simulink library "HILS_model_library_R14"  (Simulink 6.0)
undefined symbols (not defined in the file or in its folder): hilsmdl
libraries: simulink x47, simulink_extras x9, HILS_model_library x3
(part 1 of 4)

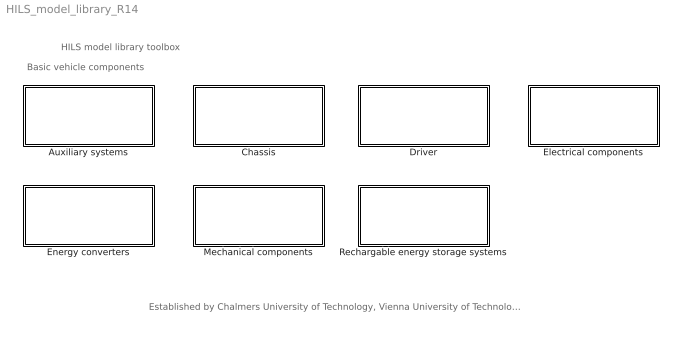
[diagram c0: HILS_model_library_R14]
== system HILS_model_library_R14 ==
  note: HILS model library toolbox
  note: Basic vehicle components
  note: Established by Chalmers University of Technology, Vienna University of Technology, Graz University of Technology, 2014
  Auxiliary systems : Subsystem
  Chassis : Subsystem
  Driver : Subsystem
  Electrical components : Subsystem
  Energy converters : Subsystem
  Mechanical components : Subsystem
  Rechargable energy storage systems : Subsystem

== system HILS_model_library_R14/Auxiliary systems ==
  Electrical auxiliary system : Subsystem
  Mechanical auxiliary system : Subsystem  mask{dat=hilsmdl.mechaux}
      mask prompts: dat "Elmotor parameter data name [struct]"

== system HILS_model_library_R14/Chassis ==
  Chassis : Subsystem  mask{dat=hilsmdl.chassis}
      mask prompts: dat "Chassis system parameter name [struct]"

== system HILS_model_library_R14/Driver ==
  Gearshift logics for manual transmission : Subsystem  mask{dat=hilsmdl.drivermanual.gearshiftmanual}
      mask prompts: dat "manual gearshift logics parameter name"
  Vehicle driver (Automatic) : Subsystem  mask{dat=hilsmdl.driverautomatic}
      mask prompts: dat "driver parameter name [struct]"
      mask help: Driver model
  Vehicle driver (Manual) : Subsystem  mask{dat=hilsmdl.drivermanual}
      mask prompts: dat "driver parameter name [struct]"
      mask help: Driver model
  Vehicle driver (Measured data) : Subsystem

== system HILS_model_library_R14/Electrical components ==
  DCDC converter : Subsystem  mask{dat=hilsmdl.dcdc}
      mask prompts: dat "DCDC parameter data name [struct]"

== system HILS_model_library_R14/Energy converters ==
  Electric machine : Subsystem  mask{dat=hilsmdl.elmachine}
      mask prompts: dat "Elmotor parameter data name [struct]"
  Hydraulic machine : Subsystem  mask{dat=hilsmdl.hydraulicmachine}
      mask prompts: dat "Hydraulic pump/motor parameter data [struct]"
  Internal Combustion Engine : Subsystem  mask{dat=hilsmdl.eng}
      mask prompts: dat "ICE parameter name [struct]"

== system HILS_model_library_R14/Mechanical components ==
  Clutch : Subsystem  mask{dat=hilsmdl.clutch}
      mask prompts: dat "Clutch system parameter name [struct]"
  Continuously variable transmission : Subsystem  mask{dat=hilsmdl.cvt}
      mask prompts: dat "Gearbox parameter data name [struct]"
  Final gear : Subsystem  mask{dat=hilsmdl.finalgear}
      mask prompts: dat "Mechanical gear parameter name [struct]"
  Mechanical connection : Subsystem  mask{dat=hilsmdl.mechconnection}
      mask prompts: dat "Mechanical gear parameter name [struct]"
  Retarder : Subsystem  mask{dat=hilsmdl.retarder}
      mask prompts: dat "Gearbox parameter data name [struct]"
  Spur gear : Subsystem  mask{dat=hilsmdl.spurgear}
      mask prompts: dat "Mechanical gear parameter name [struct]"
  Torque converter : Subsystem  mask{dat=hilsmdl.torqueconverter}
      mask prompts: dat "Torque converter parameter data name [struct]"
  Transmission : Subsystem  mask{dat=hilsmdl.transmission}
      mask prompts: dat "Gearbox parameter data name [struct]"

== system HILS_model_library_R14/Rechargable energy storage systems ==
  Accumulator : Subsystem  mask{dat=hilsmdl.accumulator}
      mask prompts: dat "RESS system parameter name [struct]"
  Battery : Subsystem  mask{dat=hilsmdl.battery}
      mask prompts: dat "RESS system parameter name [struct]"
  Flywheel : Subsystem  mask{dat=hilsmdl.flywheel}
      mask prompts: dat "Mechanical gear parameter name [struct]"
  Super Capacitor : Subsystem  mask{dat=hilsmdl.supercapacitor}
      mask prompts: dat "RESS system parameter name [struct]"

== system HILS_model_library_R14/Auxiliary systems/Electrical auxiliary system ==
  cmd : Inport
  elec in [V] : Inport  Port=2
  Model Info : simulink/Model-Wide Utilities/Model Info  InitialBlockCM=None  BlockCM=None  Frame=on  DisplayStringWithTags=|  HorizontalTextAlignment=Left  LeftAlignmentValue=0.02  SourceBlockDiagram=HILS_model_library_R14  TagMaxNumber=20
      | This model level is fixed. Place parameters in the
      | system mask on the top level. The parameter is
      | a structure specified according to GTR No XXX.
  auxiliary system : Subsystem
  local controller : Subsystem
  sensor : Outport
  elec fb out [A] : Outport  Port=2
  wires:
  local controller/1(sensor out) -> sensor/1
  auxiliary system/2(el fb out [A]) -> elec fb out [A]/1
  cmd/1 -> local controller/1(cmd in)
  elec in [V]/1 -> auxiliary system/2(el in [V])
  auxiliary system/1(sensor out) -> local controller/2(sensor in)
  local controller/2(ctrl out) -> auxiliary system/1(ctrl in)

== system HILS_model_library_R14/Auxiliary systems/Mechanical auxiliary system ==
  cmd : Inport
  mech fb in [rad/s] : Inport  Port=2
  Model Info : simulink/Model-Wide Utilities/Model Info  InitialBlockCM=None  BlockCM=None  Frame=on  DisplayStringWithTags=|  HorizontalTextAlignment=Left  LeftAlignmentValue=0.02  SourceBlockDiagram=HILS_model_library_R14  TagMaxNumber=20
      | This model level is fixed. Place parameters in the
      | system mask on the top level. The parameter is
      | a structure specified according to GTR No XXX.
  auxiliary system : Subsystem
  local controller : Subsystem
  sensor : Outport
  mech out [Nm] : Outport  Port=2
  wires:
  local controller/2(ctrl out) -> auxiliary system/1(ctrl in)
  auxiliary system/1(sensor out) -> local controller/2(sensor in)
  mech fb in [rad/s]/1 -> auxiliary system/2(mech fb in [rad/s])
  cmd/1 -> local controller/1(cmd in)
  auxiliary system/2(mech out [Nm]) -> mech out [Nm]/1
  local controller/1(sensor out) -> sensor/1

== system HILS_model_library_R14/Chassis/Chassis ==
  cmd : Inport
  mech in [Nm] : Inport  Port=2
  Model Info : simulink/Model-Wide Utilities/Model Info  InitialBlockCM=None  BlockCM=None  Frame=on  DisplayStringWithTags=|  HorizontalTextAlignment=Left  LeftAlignmentValue=0.02  SourceBlockDiagram=HILS_model_library_R14  TagMaxNumber=20
      | This model level is fixed. Place parameters in the
      | system mask on the top level. The parameter is
      | a structure specified according to GTR No XXX.
  chassis : Subsystem
  local controller : Subsystem
  sensor : Outport
  mech fb out [rad/s] : Outport  Port=2
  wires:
  cmd/1 -> local controller/1(cmd in)
  local controller/1(sensor out) -> sensor/1
  chassis/1(sensor out) -> local controller/2(sensor in)
  mech in [Nm]/1 -> chassis/2(mech in [Nm])
  chassis/2(mech fb out [rad/s]) -> mech fb out [rad/s]/1
  local controller/2(ctrl) -> chassis/1(ctrl)

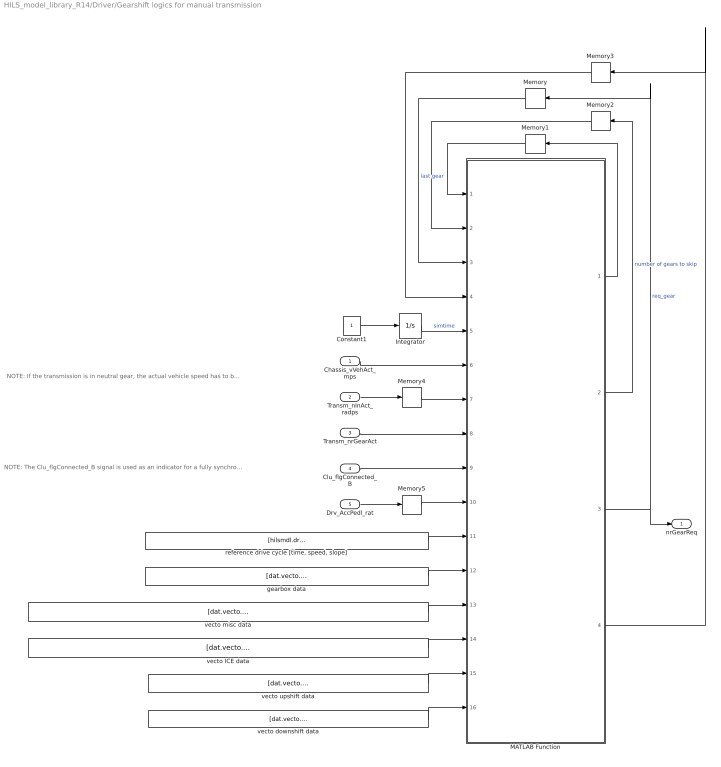
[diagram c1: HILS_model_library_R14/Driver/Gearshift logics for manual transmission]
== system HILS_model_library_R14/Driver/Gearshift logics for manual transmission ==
  note: NOTE: If the transmission is in neutral gear, the actual vehicle speed has to be zero (no rolling of the vehicle, application of brake necessary) for a correct engagement of the starting gear. Otherwise a time delay can occur until the starting gear is engaged.
  note: NOTE: The Clu_flgConnected_B signal is used as an indicator for a fully synchronized and connected drivetrain. It is involved in triggering upcoming gear shift events. Ensure that this signal becomes active only if the entire drivetrain runs on fully synchronized speeds.
  Chassis_vVehAct_mps : Inport
  Transm_nInAct_radps : Inport  Port=2
  Transm_nrGearAct : Inport  Port=3
  Clu_flgConnected_B : Inport  Port=4
  Drv_AccPedl_rat : Inport  Port=5
  Constant1 : Constant
  Integrator : Integrator
  MATLAB Function : Stateflow chart  TreatAsAtomicUnit=on
  Memory{,1..3} (4 alike) : Memory  Orientation=left
  Memory4 : Memory
  Memory5 : Memory
  gearbox data : Constant  Value=[dat.vecto.gear.number.vec; dat.vecto.gear.ratio.vec; dat.vecto.gear.efficiency.vec]
  "reference drive cycle [time, speed, slope]" : Constant  Value=[hilsmdl.drivecycle.time.vec, hilsmdl.drivecycle.speed.vec,hilsmdl.drivecycle.slope.vec]
  vecto ICE data : Constant  Value=[dat.vecto.ICE.maxtorque_speed.vec; dat.vecto.ICE.maxtorque_torque.vec; dat.vecto.ICE.maxtorque_friction.vec]
  vecto downshift data : Constant  Value=[dat.vecto.downshift_torque.vec; dat.vecto.downshift_speed.vec]
  vecto misc data : Constant  Value=[dat.vecto.vehicle.mass.value, dat.vecto.fg.ratio.value, 0.95, dat.vecto.wheel.radius.value, dat.vecto.wheel.inertia.value, dat.vecto.wheel.rollingres.value, dat.vecto.aero.af.value, dat.vecto.aero.cd.value, 80, dat.vecto.ICE.ratedspeed.value, 30, 3, dat.vecto.clutchtime.value,dat.vecto.skipgears.value,30,dat.vecto.startgearengaged.value,dat.vecto.startgearactive.value]  VectorParams1D=off
  vecto upshift data : Constant  Value=[dat.vecto.upshift_torque.vec; dat.vecto.upshift_speed.vec]
  nrGearReq : Outport
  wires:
  Constant1/1 -> Integrator/1
  Chassis_vVehAct_mps/1 -> MATLAB Function/6(act_vehicle_speed)
  MATLAB Function/3(req_gear) -> Memory/1, nrGearReq/1  "req_gear"
  "reference drive cycle [time, speed, slope]"/1 -> MATLAB Function/11(ref_drive_cycle)
  Integrator/1 -> MATLAB Function/5(simtime)  "simtime"
  Memory/1 -> MATLAB Function/3(last_req_gear)  "last gear"
  Clu_flgConnected_B/1 -> MATLAB Function/9(clutches_locked)
  Memory1/1 -> MATLAB Function/1(indicator_in)
  Transm_nInAct_radps/1 -> Memory4/1
  vecto misc data/1 -> MATLAB Function/13(VectoMisc)
  gearbox data/1 -> MATLAB Function/12(gbx)
  vecto upshift data/1 -> MATLAB Function/15(VectoShiftUp)
  MATLAB Function/2(skip_nr) -> Memory2/1  "number of gears to skip"
  Memory2/1 -> MATLAB Function/2(skip_nr_in)
  vecto ICE data/1 -> MATLAB Function/14(VectoICE)
  vecto downshift data/1 -> MATLAB Function/16(VectoShiftDown)
  MATLAB Function/1(indicator) -> Memory1/1
  MATLAB Function/4(simtime_prev_out) -> Memory3/1
  Memory3/1 -> MATLAB Function/4(simtime_prev)
  Transm_nrGearAct/1 -> MATLAB Function/8(act_gear)
  Memory4/1 -> MATLAB Function/7(act_rotational_speed)
  Drv_AccPedl_rat/1 -> Memory5/1
  Memory5/1 -> MATLAB Function/10(acc_pedal)

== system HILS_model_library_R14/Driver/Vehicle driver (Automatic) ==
  sensor in : Inport
  Bus Creator3 : BusCreator  Inputs=5
  Bus Selector1 : BusSelector  OutputSignals=Chassis.Chassis_vVehAct_mps
  Driver RefSpeed : Subsystem
  Ground : Ground
  Ground1 : Ground
  driver cmd out : Outport
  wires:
  Ground1/1 -> Bus Creator3/5  "Drv_CluPedl_Rt"
  Ground/1 -> Bus Creator3/4  "Drv_nrGearReq"
  Bus Selector1/1 -> Driver RefSpeed/1(Chassis_vVehAct_mps)  "<Chassis_vVehAct_mps>"
  Driver RefSpeed/1(CycleReferenceSpeed_mps) -> Bus Creator3/1  "Drivecycle_RefSpeed_mps"
  Driver RefSpeed/2(Drv_BrkPedl_rat) -> Bus Creator3/2  "Drv_BrkPedl_Rt"
  Driver RefSpeed/3(Drv_AccPedl_rat) -> Bus Creator3/3  "Drv_AccPedl_Rt"
  sensor in/1 -> Bus Selector1/1
  Bus Creator3/1 -> driver cmd out/1  "Driver"

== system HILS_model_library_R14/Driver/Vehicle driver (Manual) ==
  note: NOTE: The Clu_flgConnected_B signal is used as an indicator for a fully synchronized and connected drivetrain. It is involved in triggering upcoming gear shift events. Ensure that this signal becomes active only if the entire drivetrain runs on fully synchronized speeds.
  sensor in : Inport
  Bus Creator3 : BusCreator  Inputs=5
  Bus Selector1 : BusSelector  OutputSignals=Chassis.Chassis_vVehAct_mps,Transmission.Transm_nInAct_radps,Transmission.Transm_nrGearAct,Clutch.Clu_flgConnected_B,Driver.Drv_AccPedl_Rt
  Clutch actuator : Subsystem
  Data Type Conversion : DataTypeConversion
  Driver RefSpeed : Subsystem
  Gearshift logics for manual transmission : HILS_model_library/Driver/Gearshift logics for manual transmission  dat=hilsmdl.drivermanual.gearshiftmanual
  driver cmd out : Outport
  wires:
  Bus Selector1/5 -> Gearshift logics for manual transmission/5  "<Drv_AccPedl_Rt>"
  Clutch actuator/1(DrvResetAndHoldZero) -> Driver RefSpeed/2(AccPdlResetAndHoldZero)  "DrvResetAndHoldZero"
  Clutch actuator/2(Drv_gearReq_out) -> Bus Creator3/4  "Drv_nrGearReq"
  Clutch actuator/3(DrvReqClu) -> Bus Creator3/5  "Drv_CluPedl_Rt"
  Bus Selector1/2 -> Gearshift logics for manual transmission/2  "<Transm_nInAct_radps>"
  Bus Selector1/1 -> Gearshift logics for manual transmission/1, Driver RefSpeed/1(Chassis_vVehAct_mps)  "<Chassis_vVehAct_mps>"
  Bus Selector1/4 -> Gearshift logics for manual transmission/4, Data Type Conversion/1  "<Clu_flgConnected_B>"
  Bus Selector1/3 -> Gearshift logics for manual transmission/3  "<Transm_nrGearAct>"
  Data Type Conversion/1 -> Clutch actuator/3(releaseDrvResetAndHoldZero)
  Gearshift logics for manual transmission/1 -> Clutch actuator/2(Drv_gearReq)  "Drv_gearReq"
  Driver RefSpeed/1(CycleReferenceSpeed_mps) -> Bus Creator3/1  "Drivecycle_RefSpeed_mps"
  Driver RefSpeed/2(Drv_BrkPedl_rat) -> Bus Creator3/2  "Drv_BrkPedl_Rt"
  Driver RefSpeed/3(Drv_AccPedl_rat) -> Bus Creator3/3, Clutch actuator/1(Drv_AccPedl_rat)  "Drv_AccPedl_Rt"
  sensor in/1 -> Bus Selector1/1
  Bus Creator3/1 -> driver cmd out/1  "Driver"

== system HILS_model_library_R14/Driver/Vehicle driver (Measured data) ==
  sensor in : Inport
  Bus Creator3 : BusCreator  Inputs=5
  From Workspace : FromWorkspace  VariableName=certmdl_input.Drv_BrkPedl_rat  SampleTime=0
  From Workspace1 : FromWorkspace  VariableName=certmdl_input.Drv_AccPedl_rat  SampleTime=0
  Ground : Ground
  Ground1 : Ground
  Ground2 : Ground
  Terminator : Terminator
  driver cmd out : Outport
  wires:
  Bus Creator3/1 -> driver cmd out/1  "Driver"
  From Workspace1/1 -> Bus Creator3/3  "Drv_AccPedl_Rt"
  From Workspace/1 -> Bus Creator3/2  "Drv_BrkPedl_Rt"
  Ground2/1 -> Bus Creator3/1  "Drivecycle_RefSpeed_mps"
  Ground/1 -> Bus Creator3/4  "Drv_nrGearReq"
  Ground1/1 -> Bus Creator3/5  "Drv_CluPedl_Rt"
  sensor in/1 -> Terminator/1

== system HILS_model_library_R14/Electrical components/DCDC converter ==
  cmd : Inport
  elec in [V] : Inport  Port=2
  elec fb in [A] : Inport  Port=3
  Converter : Subsystem
  Model Info : simulink/Model-Wide Utilities/Model Info  InitialBlockCM=None  BlockCM=None  Frame=on  DisplayStringWithTags=|  HorizontalTextAlignment=Left  LeftAlignmentValue=0.02  SourceBlockDiagram=HILS_model_library_R14  TagMaxNumber=20
      | This model level is fixed. Place parameters in the
      | system mask on the top level. The parameter is
      | a structure specified according to GTR No XXX.
  local controller : Subsystem
  sensor : Outport
  elec out [V] : Outport  Port=2
  elec fb out [A] : Outport  Port=3
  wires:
  elec fb in [A]/1 -> Converter/3(elec fb in [A])
  Converter/2(elec out [V]) -> elec out [V]/1
  elec in [V]/1 -> Converter/2(elec in [V])
  Converter/3(elec fb out [A]) -> elec fb out [A]/1
  cmd/1 -> local controller/1(cmd)
  local controller/2(ctrl) -> Converter/1(ctrl)
  local controller/1(sensor out) -> sensor/1
  Converter/1(Sensor) -> local controller/2(sensor in)

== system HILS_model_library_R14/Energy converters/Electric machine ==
  cmd : Inport
  elec in [V] : Inport  Port=2
  mech fb in [rad/s] : Inport  Port=3
  Model Info : simulink/Model-Wide Utilities/Model Info  InitialBlockCM=None  BlockCM=None  Frame=on  DisplayStringWithTags=|  HorizontalTextAlignment=Left  LeftAlignmentValue=0.02  SourceBlockDiagram=HILS_model_library_R14  TagMaxNumber=20
      | This model level is fixed. Place parameters in the
      | system mask on the top level. The parameter is
      | a structure specified according to GTR No XXX.
  electric machine : Subsystem
  local controller : Subsystem
  sensor : Outport
  mech out [Nm] : Outport  Port=2
  elec fb out [A] : Outport  Port=3
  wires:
  local controller/2(ctrl out) -> electric machine/1(ctrl in)
  electric machine/1(sensor out) -> local controller/2(sensor in)
  elec in [V]/1 -> electric machine/2(el in [V])
  mech fb in [rad/s]/1 -> electric machine/3(mech fb in [rad/s])
  cmd/1 -> local controller/1(cmd in)
  electric machine/3(el fb out [A]) -> elec fb out [A]/1
  electric machine/2(mech out [Nm]) -> mech out [Nm]/1
  local controller/1(sensor out) -> sensor/1

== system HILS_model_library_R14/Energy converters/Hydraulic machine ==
  cmd : Inport
  fluid in 1 [Pa] : Inport  Port=2
  fluid in 2 [Pa] : Inport  Port=3
  mech fb in [rad/s] : Inport  Port=4
  hydraulic machine : Subsystem
  local controller : Subsystem
  sensor : Outport
  mech out [Nm] : Outport  Port=2
  fluid fb out [m3/s] : Outport  Port=3
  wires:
  local controller/1(sensor out) -> sensor/1
  hydraulic machine/2(mech power out [Nm]) -> mech out [Nm]/1
  hydraulic machine/3(flow fb out [m3/s]) -> fluid fb out [m3/s]/1
  cmd/1 -> local controller/1(cmd in)
  fluid in 2 [Pa]/1 -> hydraulic machine/3(res pressure in [Pa])
  fluid in 1 [Pa]/1 -> hydraulic machine/2(acc pressure in [Pa])
  hydraulic machine/1(sensor out) -> local controller/2(sensor in)
  local controller/2(ctrl out) -> hydraulic machine/1(ctrl in)
  mech fb in [rad/s]/1 -> hydraulic machine/4(mech fb in [rad/s])

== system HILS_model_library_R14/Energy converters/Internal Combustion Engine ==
  cmd : Inport
  mech fb in [rad/s] : Inport  Port=2
  Engine model : Subsystem
  Model Info : simulink/Model-Wide Utilities/Model Info  InitialBlockCM=None  BlockCM=None  Frame=on  DisplayStringWithTags=|  HorizontalTextAlignment=Left  LeftAlignmentValue=0.02  SourceBlockDiagram=HILS_model_library_R14  TagMaxNumber=20
      | This model level is fixed. Place parameters in the
      | system mask on the top level. The parameter is
      | a structure specified according to GTR No XXX.
  local controller : Subsystem
  sensor : Outport
  mech out [Nm] : Outport  Port=2
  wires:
  local controller/1(sensor) -> sensor/1
  Engine model/2(mech power out [Nm]) -> mech out [Nm]/1
  cmd/1 -> local controller/1(cmd in)
  mech fb in [rad/s]/1 -> Engine model/2(mech fb in [rad/s])
  Engine model/1(sensor out) -> local controller/2(sensor in)
  local controller/2(ctrl out) -> Engine model/1(ctrl in)

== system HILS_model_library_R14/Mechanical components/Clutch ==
  cmd : Inport
  mech in [Nm] : Inport  Port=2
  mech fb in [rad/s] : Inport  Port=3
  Clutch : Subsystem
  Model Info : simulink/Model-Wide Utilities/Model Info  InitialBlockCM=None  BlockCM=None  Frame=on  DisplayStringWithTags=|  HorizontalTextAlignment=Left  LeftAlignmentValue=0.02  SourceBlockDiagram=HILS_model_library_R14  TagMaxNumber=20
      | This model level is fixed. Place parameters in the
      | system mask on the top level. The parameter is
      | a structure specified according to GTR No XXX.
  local controller : Subsystem
  sensor : Outport
  mech out [Nm] : Outport  Port=2
  mech fb out [rad/s] : Outport  Port=3
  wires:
  local controller/1(sensor) -> sensor/1
  local controller/2(ctrl) -> Clutch/1(ctrl)
  Clutch/1(sensor out) -> local controller/2(sensor in)
  cmd/1 -> local controller/1(cmd in)
  Clutch/3(mech fb out [rad/s]) -> mech fb out [rad/s]/1
  mech fb in [rad/s]/1 -> Clutch/3(mech fb in [rad/s])
  Clutch/2(mech out [Nm]) -> mech out [Nm]/1
  mech in [Nm]/1 -> Clutch/2(mech in [Nm])

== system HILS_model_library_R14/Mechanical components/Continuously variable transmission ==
  cmd : Inport
  mech in [Nm] : Inport  Port=2
  mech fb in [rad/s] : Inport  Port=3
  Model Info : simulink/Model-Wide Utilities/Model Info  InitialBlockCM=None  BlockCM=None  Frame=on  DisplayStringWithTags=|  HorizontalTextAlignment=Left  LeftAlignmentValue=0.02  SourceBlockDiagram=HILS_model_library_R14  TagMaxNumber=20
      | This model level is fixed. Place parameters in the
      | system mask on the top level. The parameter is
      | a structure specified according to GTR No XXX.
  Transmission : Subsystem
  local controller : Subsystem
  sensor : Outport
  mech out [Nm] : Outport  Port=2
  mech fb out [rad/s] : Outport  Port=3
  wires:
  mech fb in [rad/s]/1 -> Transmission/3(mech fb in [rad/s])
  Transmission/2(mech out [Nm]) -> mech out [Nm]/1
  mech in [Nm]/1 -> Transmission/2(mech in [Nm])
  Transmission/3(mech fb out [rad/s]) -> mech fb out [rad/s]/1
  cmd/1 -> local controller/1(cmd)
  local controller/2(ctrl) -> Transmission/1(ctrl)
  local controller/1(sensor out) -> sensor/1
  Transmission/1(Out1) -> local controller/2(sensor in)

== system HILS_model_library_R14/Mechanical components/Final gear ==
  mech in [Nm] : Inport
  mech fb in [rad/s] : Inport  Port=2
  2-D Lookup Table : Lookup_n-D  BreakpointsForDimension1=dat.mechefficiency.torque.vec  BreakpointsForDimension2=dat.mechefficiency.speed.vec  Table=dat.mechefficiency.efficiency.map  ExtrapMethod=None - Clip
  Abs : Abs
  Bus Creator : BusCreator  Inputs=1
  Bus Creator1 : BusCreator  Inputs=2
  Bus Selector1 : BusSelector  OutputSignals=phys_speed_radps
  Bus Selector5 : BusSelector  OutputSignals=phys_torque_Nm,phys_inertia_kgm2
  Constant : Constant  Value=dat.inertia.value
  Fcn : Fcn  Expr=1/u(1)
  Memory : Memory
  Model Info : simulink/Model-Wide Utilities/Model Info  InitialBlockCM=None  BlockCM=None  Frame=on  DisplayStringWithTags=|  HorizontalTextAlignment=Left  LeftAlignmentValue=0.02  SourceBlockDiagram=HILS_model_library_R14  TagMaxNumber=20
      | This model level is fixed. Place parameters in the
      | system mask on the top level. The parameter is
      | a structure specified according to GTR No XXX.
  Product : Product
  Sum3 : Sum  Inputs=|++
  Switch : Switch
  gear ratio : Gain  Gain=dat.ratio.value
  gear ratio1 : Gain  Gain=dat.ratio.value
  gear ratio5 : Gain  Gain=dat.ratio.value^2
  mech out [Nm] : Outport
  mech fb out [rad/s] : Outport  Port=2
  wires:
  Product/1 -> Bus Creator1/1  "phys_torque_Nm"
  Constant/1 -> Sum3/2
  Sum3/1 -> gear ratio5/1
  Bus Selector5/2 -> Sum3/1  "<phys_inertia_kgm2>"
  gear ratio/1 -> Memory/1, Bus Creator/1  "phys_speed_radps"
  gear ratio5/1 -> Bus Creator1/2  "phys_inertia_kgm2"
  Bus Selector5/1 -> gear ratio1/1, Switch/2, Abs/1  "<phys_torque_Nm>"
  Bus Creator1/1 -> mech out [Nm]/1
  Bus Creator/1 -> mech fb out [rad/s]/1
  mech in [Nm]/1 -> Bus Selector5/1
  Bus Selector1/1 -> gear ratio/1  "<phys_speed_radps>"
  mech fb in [rad/s]/1 -> Bus Selector1/1
  2-D Lookup Table/1 -> Switch/1, Fcn/1  "efficiency"
  gear ratio1/1 -> Product/1
  Switch/1 -> Product/2
  Abs/1 -> 2-D Lookup Table/1
  Fcn/1 -> Switch/3
  Memory/1 -> 2-D Lookup Table/2

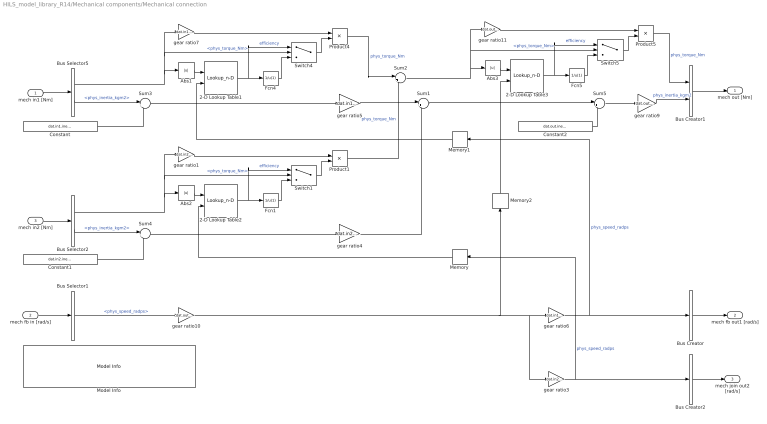
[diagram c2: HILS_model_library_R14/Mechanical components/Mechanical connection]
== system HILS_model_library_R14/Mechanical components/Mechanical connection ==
  mech in1 [Nm] : Inport
  mech fb in [rad/s] : Inport  Port=2
  mech in2 [Nm] : Inport  Port=3
  2-D Lookup Table1 : Lookup_n-D  BreakpointsForDimension1=dat.in1.mechefficiency.torque.vec  BreakpointsForDimension2=dat.in1.mechefficiency.speed.vec  Table=dat.in1.mechefficiency.efficiency.map  ExtrapMethod=None - Clip
  2-D Lookup Table2 : Lookup_n-D  BreakpointsForDimension1=dat.in2.mechefficiency.torque.vec  BreakpointsForDimension2=dat.in2.mechefficiency.speed.vec  Table=dat.in2.mechefficiency.efficiency.map  ExtrapMethod=None - Clip
  2-D Lookup Table3 : Lookup_n-D  BreakpointsForDimension1=dat.out.mechefficiency.torque.vec  BreakpointsForDimension2=dat.out.mechefficiency.speed.vec  Table=dat.out.mechefficiency.efficiency.map  ExtrapMethod=None - Clip
  Abs1 : Abs
  Abs2 : Abs
  Abs3 : Abs
  Bus Creator : BusCreator  Inputs=1
  Bus Creator1 : BusCreator  Inputs=2
  Bus Creator2 : BusCreator  Inputs=1
  Bus Selector1 : BusSelector  OutputSignals=phys_speed_radps
  Bus Selector2 : BusSelector  OutputSignals=phys_torque_Nm,phys_inertia_kgm2
  Bus Selector5 : BusSelector  OutputSignals=phys_torque_Nm,phys_inertia_kgm2
  Constant : Constant  Value=dat.in1.inertia.value
  Constant1 : Constant  Value=dat.in2.inertia.value
  Constant2 : Constant  Value=dat.out.inertia.value
  Fcn1 : Fcn  Expr=1/u(1)
  Fcn4 : Fcn  Expr=1/u(1)
  Fcn5 : Fcn  Expr=1/u(1)
  Memory : Memory  Orientation=left
  Memory1 : Memory  Orientation=left
  Memory2 : Memory  Orientation=up
  Model Info : simulink/Model-Wide Utilities/Model Info  InitialBlockCM=None  BlockCM=None  Frame=on  DisplayStringWithTags=|  HorizontalTextAlignment=Left  LeftAlignmentValue=0.02  SourceBlockDiagram=HILS_model_library_R14  TagMaxNumber=20
      | This model level is fixed. Place parameters in the
      | system mask on the top level. The parameter is
      | a structure specified according to GTR No XXX.
  Product1 : Product
  Product4 : Product
  Product5 : Product
  Sum{1..5} (5 alike) : Sum  Inputs=|++
  Switch1 : Switch
  Switch4 : Switch
  Switch5 : Switch
  gear ratio1 : Gain  Gain=dat.in2.ratio.value
  gear ratio10 : Gain  Gain=dat.out.ratio.value
  gear ratio11 : Gain  Gain=dat.out.ratio.value
  gear ratio3 : Gain  Gain=dat.in2.ratio.value
  gear ratio4 : Gain  Gain=dat.in2.ratio.value^2
  gear ratio5 : Gain  Gain=dat.in1.ratio.value^2
  gear ratio6 : Gain  Gain=dat.in1.ratio.value
  gear ratio7 : Gain  Gain=dat.in1.ratio.value
  gear ratio9 : Gain  Gain=dat.out.ratio.value^2
  mech out [Nm] : Outport
  mech fb out1 [rad/s] : Outport  Port=2
  mech join out2 [rad/s] : Outport  Port=3
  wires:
  Constant2/1 -> Sum5/2
  Sum1/1 -> Sum5/1
  Sum5/1 -> gear ratio9/1
  Bus Selector2/2 -> Sum4/1  "<phys_inertia_kgm2>"
  Constant1/1 -> Sum4/2
  Sum4/1 -> gear ratio4/1
  Constant/1 -> Sum3/2
  Sum3/1 -> gear ratio5/1
  Bus Selector5/2 -> Sum3/1  "<phys_inertia_kgm2>"
  gear ratio9/1 -> Bus Creator1/2  "phys_inertia_kgm2"
  gear ratio5/1 -> Sum1/1
  Bus Creator1/1 -> mech out [Nm]/1
  Bus Creator/1 -> mech fb out1 [rad/s]/1
  mech in1 [Nm]/1 -> Bus Selector5/1
  Bus Selector1/1 -> gear ratio10/1  "<phys_speed_radps>"
  mech fb in [rad/s]/1 -> Bus Selector1/1
  Bus Selector2/1 -> gear ratio1/1, Switch1/2, Abs2/1  "<phys_torque_Nm>"
  Bus Creator2/1 -> mech join out2 [rad/s]/1
  mech in2 [Nm]/1 -> Bus Selector2/1
  gear ratio4/1 -> Sum1/2
  gear ratio3/1 -> Memory/1, Bus Creator2/1  "phys_speed_radps"
  gear ratio7/1 -> Product4/1
  Product4/1 -> Sum2/1  "phys_torque_Nm"
  gear ratio6/1 -> Memory1/1, Bus Creator/1  "phys_speed_radps"
  Bus Selector5/1 -> gear ratio7/1, Switch4/2, Abs1/1  "<phys_torque_Nm>"
  2-D Lookup Table1/1 -> Switch4/1, Fcn4/1  "efficiency"
  Switch4/1 -> Product4/2
  Abs1/1 -> 2-D Lookup Table1/1
  Fcn4/1 -> Switch4/3
  gear ratio1/1 -> Product1/1
  Product1/1 -> Sum2/2  "phys_torque_Nm"
  2-D Lookup Table2/1 -> Switch1/1, Fcn1/1  "efficiency"
  Switch1/1 -> Product1/2
  Abs2/1 -> 2-D Lookup Table2/1
  Fcn1/1 -> Switch1/3
  Sum2/1 -> gear ratio11/1, Switch5/2, Abs3/1  "<phys_torque_Nm>"
  gear ratio11/1 -> Product5/1
  Product5/1 -> Bus Creator1/1  "phys_torque_Nm"
  2-D Lookup Table3/1 -> Switch5/1, Fcn5/1  "efficiency"
  Switch5/1 -> Product5/2
  Abs3/1 -> 2-D Lookup Table3/1
  Fcn5/1 -> Switch5/3
  gear ratio10/1 -> Memory2/1, gear ratio6/1, gear ratio3/1
  Memory/1 -> 2-D Lookup Table2/2
  Memory1/1 -> 2-D Lookup Table1/2
  Memory2/1 -> 2-D Lookup Table3/2

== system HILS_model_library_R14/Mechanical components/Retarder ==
  cmd : Inport
  mech in [Nm] : Inport  Port=2
  mech fb in [rad/s] : Inport  Port=3
  Model Info : simulink/Model-Wide Utilities/Model Info  InitialBlockCM=None  BlockCM=None  Frame=on  DisplayStringWithTags=|  HorizontalTextAlignment=Left  LeftAlignmentValue=0.02  SourceBlockDiagram=HILS_model_library_R14  TagMaxNumber=20
      | This model level is fixed. Place parameters in the
      | system mask on the top level. The parameter is
      | a structure specified according to GTR No XXX.
  Retarder : Subsystem
  local controller : Subsystem
  sensor : Outport
  mech out [Nm] : Outport  Port=2
  mech fb out [rad/s] : Outport  Port=3
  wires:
  Retarder/1(Out1) -> local controller/2(sensor in)
  local controller/1(sensor out) -> sensor/1
  local controller/2(ctrl) -> Retarder/1(ctrl)
  cmd/1 -> local controller/1(cmd)
  Retarder/3(mech fb out [rad/s]) -> mech fb out [rad/s]/1
  mech in [Nm]/1 -> Retarder/2(mech in [Nm])
  Retarder/2(mech out [Nm]) -> mech out [Nm]/1
  mech fb in [rad/s]/1 -> Retarder/3(mech fb in [rad/s])

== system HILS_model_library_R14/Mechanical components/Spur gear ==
  mech in [Nm] : Inport
  mech fb in [rad/s] : Inport  Port=2
  2-D Lookup Table : Lookup_n-D  BreakpointsForDimension1=dat.mechefficiency.torque.vec  BreakpointsForDimension2=dat.mechefficiency.speed.vec  Table=dat.mechefficiency.efficiency.map  ExtrapMethod=None - Clip
  Abs : Abs
  Bus Creator : BusCreator  Inputs=1
  Bus Creator1 : BusCreator  Inputs=2
  Bus Selector1 : BusSelector  OutputSignals=phys_speed_radps
  Bus Selector5 : BusSelector  OutputSignals=phys_torque_Nm,phys_inertia_kgm2
  Constant : Constant  Value=dat.inertia.value
  Fcn1 : Fcn  Expr=1/u(1)
  Memory : Memory
  Model Info : simulink/Model-Wide Utilities/Model Info  InitialBlockCM=None  BlockCM=None  Frame=on  DisplayStringWithTags=|  HorizontalTextAlignment=Left  LeftAlignmentValue=0.02  SourceBlockDiagram=HILS_model_library_R14  TagMaxNumber=20
      | This model level is fixed. Place parameters in the
      | system mask on the top level. The parameter is
      | a structure specified according to GTR No XXX.
  Product : Product
  Sum3 : Sum  Inputs=|++
  Switch1 : Switch
  gear ratio1 : Gain  Gain=dat.ratio.value
  gear ratio10 : Gain  Gain=dat.ratio.value
  gear ratio5 : Gain  Gain=dat.ratio.value^2
  mech out [Nm] : Outport
  mech fb out [rad/s] : Outport  Port=2
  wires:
  mech fb in [rad/s]/1 -> Bus Selector1/1
  Bus Selector1/1 -> gear ratio10/1  "<phys_speed_radps>"
  mech in [Nm]/1 -> Bus Selector5/1
  Bus Creator/1 -> mech fb out [rad/s]/1
  Bus Creator1/1 -> mech out [Nm]/1
  gear ratio5/1 -> Bus Creator1/2  "phys_inertia_kgm2"
  Bus Selector5/2 -> Sum3/1  "<phys_inertia_kgm2>"
  Sum3/1 -> gear ratio5/1
  Constant/1 -> Sum3/2
  gear ratio1/1 -> Product/1
  Product/1 -> Bus Creator1/1  "phys_torque_Nm"
  gear ratio10/1 -> Memory/1, Bus Creator/1  "phys_speed_radps"
  Bus Selector5/1 -> Abs/1, Switch1/2, gear ratio1/1  "<phys_torque_Nm>"
  2-D Lookup Table/1 -> Switch1/1, Fcn1/1  "efficiency"
  Switch1/1 -> Product/2
  Abs/1 -> 2-D Lookup Table/1
  Fcn1/1 -> Switch1/3
  Memory/1 -> 2-D Lookup Table/2

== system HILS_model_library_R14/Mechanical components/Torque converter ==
  cmd : Inport
  mech in [Nm] : Inport  Port=2
  mech fb in [rad/s] : Inport  Port=3
  Model Info : simulink/Model-Wide Utilities/Model Info  InitialBlockCM=None  BlockCM=None  Frame=on  DisplayStringWithTags=|  HorizontalTextAlignment=Left  LeftAlignmentValue=0.02  SourceBlockDiagram=HILS_model_library_R14  TagMaxNumber=20
      | This model level is fixed. Place parameters in the
      | system mask on the top level. The parameter is
      | a structure specified according to GTR No XXX.
  Torque converter : Subsystem
  local controller : Subsystem
  sensor : Outport
  mech out [Nm] : Outport  Port=2
  mech fb out [rad/s] : Outport  Port=3
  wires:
  mech fb in [rad/s]/1 -> Torque converter/3(mech fb in [rad/s])
  Torque converter/1(mech out [Nm]) -> mech out [Nm]/1
  mech in [Nm]/1 -> Torque converter/2(mech in [Nm])
  Torque converter/2(mech fb out [rad/s]) -> mech fb out [rad/s]/1
  cmd/1 -> local controller/1(cmd)
  local controller/2(ctrl) -> Torque converter/1(ctrl)
  local controller/1(sensor out) -> sensor/1
  Torque converter/3(sensor out) -> local controller/2(sensor in)

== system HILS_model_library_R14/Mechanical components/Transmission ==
  cmd : Inport
  mech in [Nm] : Inport  Port=2
  mech fb in [rad/s] : Inport  Port=3
  Model Info : simulink/Model-Wide Utilities/Model Info  InitialBlockCM=None  BlockCM=None  Frame=on  DisplayStringWithTags=|  HorizontalTextAlignment=Left  LeftAlignmentValue=0.02  SourceBlockDiagram=HILS_model_library_R14  TagMaxNumber=20
      | This model level is fixed. Place parameters in the
      | system mask on the top level. The parameter is
      | a structure specified according to GTR No XXX.
  Transmission : Subsystem
  local controller : Subsystem
  sensor : Outport
  mech out [Nm] : Outport  Port=2
  mech fb out [rad/s] : Outport  Port=3
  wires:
  Transmission/1(Out1) -> local controller/2(sensor in)
  local controller/1(sensor out) -> sensor/1
  local controller/2(ctrl) -> Transmission/1(ctrl)
  cmd/1 -> local controller/1(cmd)
  Transmission/3(mech fb out [rad/s]) -> mech fb out [rad/s]/1
  mech in [Nm]/1 -> Transmission/2(mech in [Nm])
  Transmission/2(mech out [Nm]) -> mech out [Nm]/1
  mech fb in [rad/s]/1 -> Transmission/3(mech fb in [rad/s])

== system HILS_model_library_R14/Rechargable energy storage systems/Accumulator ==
  cmd : Inport
  fluid fb in [m3/s] : Inport  Port=2
  Model Info1 : simulink/Model-Wide Utilities/Model Info  InitialBlockCM=None  BlockCM=None  Frame=on  DisplayStringWithTags=|  HorizontalTextAlignment=Left  LeftAlignmentValue=0.02  SourceBlockDiagram=HILS_model_library_R14  TagMaxNumber=20
      | This model level is fixed. Place parameters in the
      | system mask on the top level. The parameter is
      | a structure specified according to GTR No XXX.
  local controller : Subsystem
  tank : Subsystem
  sensor : Outport
  fluid out [Pa] : Outport  Port=2
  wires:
  cmd/1 -> local controller/1(cmd in)
  tank/1(sensor out) -> local controller/2(sensor in)
  fluid fb in [m3/s]/1 -> tank/2(flow fb in [m3/s])
  local controller/1(sensor) -> sensor/1
  tank/2(pressure out [Pa]) -> fluid out [Pa]/1
  local controller/2(ctrl) -> tank/1(flow fb in [m3/s]1)

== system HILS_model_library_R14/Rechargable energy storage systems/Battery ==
  cmd : Inport
  elec fb in [A] : Inport  Port=2
  Battery model : Subsystem
  Model Info1 : simulink/Model-Wide Utilities/Model Info  InitialBlockCM=None  BlockCM=None  Frame=on  DisplayStringWithTags=|  HorizontalTextAlignment=Left  LeftAlignmentValue=0.02  SourceBlockDiagram=HILS_model_library_R14  TagMaxNumber=20
      | This model level is fixed. Place parameters in the
      | system mask on the top level. The parameter is
      | a structure specified according to GTR No XXX.
  local controller : Subsystem
  sensor : Outport
  elec out [V] : Outport  Port=2
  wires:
  Battery model/2(el out [V]) -> elec out [V]/1
  local controller/1(sensor) -> sensor/1
  elec fb in [A]/1 -> Battery model/2(el fb in [A])
  Battery model/1(sensor out) -> local controller/2(sensor in)
  local controller/2(ctrl out) -> Battery model/1(ctrl in)
  cmd/1 -> local controller/1(cmd in)

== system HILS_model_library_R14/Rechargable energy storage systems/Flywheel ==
  cmd : Inport
  mech in [Nm] : Inport  Port=2
  Model Info : simulink/Model-Wide Utilities/Model Info  InitialBlockCM=None  BlockCM=None  Frame=on  DisplayStringWithTags=|  HorizontalTextAlignment=Left  LeftAlignmentValue=0.02  SourceBlockDiagram=HILS_model_library_R14  TagMaxNumber=20
      | This model level is fixed. Place parameters in the
      | system mask on the top level. The parameter is
      | a structure specified according to GTR No XXX.
  flywheel model : Subsystem
  local controller : Subsystem
  sensor out : Outport
  mech fb out [rad/s] : Outport  Port=2
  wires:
  local controller/2(ctrl out) -> flywheel model/1(ctrl in)
  flywheel model/1(sensor out) -> local controller/2(sensor in)
  mech in [Nm]/1 -> flywheel model/2(mech in [Nm])
  cmd/1 -> local controller/1(cmd in)
  flywheel model/2(mech fb out [rad/s]) -> mech fb out [rad/s]/1
  local controller/1(sensor) -> sensor out/1

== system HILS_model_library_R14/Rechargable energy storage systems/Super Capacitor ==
  cmd : Inport
  elec fb in [A] : Inport  Port=2
  Model Info1 : simulink/Model-Wide Utilities/Model Info  InitialBlockCM=None  BlockCM=None  Frame=on  DisplayStringWithTags=|  HorizontalTextAlignment=Left  LeftAlignmentValue=0.02  SourceBlockDiagram=HILS_model_library_R14  TagMaxNumber=20
      | This model level is fixed. Place parameters in the
      | system mask on the top level. The parameter is
      | a structure specified according to GTR No XXX.
  Supercap model : Subsystem
  local controller : Subsystem
  sensor : Outport
  elec out [V] : Outport  Port=2
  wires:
  cmd/1 -> local controller/1(cmd in)
  local controller/2(ctrl) -> Supercap model/1(ctrl)
  Supercap model/1(sensor out) -> local controller/2(sensor in)
  elec fb in [A]/1 -> Supercap model/2(el fb in [A])
  local controller/1(sensor) -> sensor/1
  Supercap model/2(el out [V]) -> elec out [V]/1

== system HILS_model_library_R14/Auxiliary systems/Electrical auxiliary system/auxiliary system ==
  ctrl in : Inport
  el in [V] : Inport  Port=2
  Bus Creator1 : BusCreator  Inputs=1
  Bus Creator2 : BusCreator  Inputs=1
  Bus Selector1 : BusSelector  OutputSignals=phys_voltage_V
  Bus Selector3 : BusSelector  OutputSignals=Aux_pwrElecReq_W
  Constant : Constant  Value=0
  Gain3 : Gain
  Product1 : Product  Inputs=*/
  Switch : Switch  Criteria=u2 ~= 0
  sensor out : Outport
  el fb out [A] : Outport  Port=2
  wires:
  Bus Selector1/1 -> Switch/2, Product1/2  "<phys_voltage_V>"
  Bus Selector3/1 -> Product1/1  "<Aux_pwrElecReq_W>"
  Bus Creator1/1 -> el fb out [A]/1
  el in [V]/1 -> Bus Selector1/1
  ctrl in/1 -> Bus Selector3/1
  Bus Creator2/1 -> sensor out/1
  Gain3/1 -> Bus Creator2/1  "Aux_iAct_A"
  Switch/1 -> Gain3/1, Bus Creator1/1  "phys_current_A"
  Constant/1 -> Switch/3
  Product1/1 -> Switch/1

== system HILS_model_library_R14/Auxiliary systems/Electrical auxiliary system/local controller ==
  cmd in : Inport
  sensor in : Inport  Port=2
  Bus Creator1 : BusCreator  Inputs=1
  Bus Creator2 : BusCreator  Inputs=1
  Bus Selector1 : BusSelector  OutputSignals=Aux_pwrElecReq_W
  Bus Selector3 : BusSelector  OutputSignals=Aux_iAct_A
  sensor out : Outport
  ctrl out : Outport  Port=2
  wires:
  Bus Selector1/1 -> Bus Creator1/1  "<Aux_pwrElecReq_W>"
  Bus Selector3/1 -> Bus Creator2/1  "<Aux_iAct_A>"
  cmd in/1 -> Bus Selector1/1
  Bus Creator2/1 -> sensor out/1  "Auxiliary"
  sensor in/1 -> Bus Selector3/1
  Bus Creator1/1 -> ctrl out/1

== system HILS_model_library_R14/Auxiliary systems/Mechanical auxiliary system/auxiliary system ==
  ctrl in : Inport
  mech fb in [rad/s] : Inport  Port=2
  Bus Creator : BusCreator  Inputs=2
  Bus Creator2 : BusCreator  Inputs=1
  Bus Selector2 : BusSelector  OutputSignals=phys_speed_radps
  Bus Selector3 : BusSelector  OutputSignals=Aux_pwrMechReq_W
  Constant : Constant  Value=0
  Constant1 : Constant  Value=dat.inertia.value
  Gain3 : Gain
  Product1 : Product  Inputs=*/
  Switch : Switch  Criteria=u2 ~= 0
  sensor out : Outport
  mech out [Nm] : Outport  Port=2
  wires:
  Constant1/1 -> Bus Creator/2  "phys_inertia_kgm2"
  Bus Selector2/1 -> Switch/2, Product1/2  "<phys_speed_radps>"
  mech fb in [rad/s]/1 -> Bus Selector2/1
  Bus Creator/1 -> mech out [Nm]/1
  Bus Selector3/1 -> Product1/1  "<Aux_pwrMechReq_W>"
  ctrl in/1 -> Bus Selector3/1
  Bus Creator2/1 -> sensor out/1
  Gain3/1 -> Bus Creator2/1  "Aux_tqAct_Nm"
  Switch/1 -> Gain3/1, Bus Creator/1  "phys_torque_Nm"
  Constant/1 -> Switch/3
  Product1/1 -> Switch/1

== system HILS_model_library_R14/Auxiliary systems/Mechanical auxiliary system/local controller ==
  cmd in : Inport
  sensor in : Inport  Port=2
  Bus Creator1 : BusCreator  Inputs=1
  Bus Creator2 : BusCreator  Inputs=1
  Bus Selector1 : BusSelector  OutputSignals=Aux_pwrMechReq_W
  Bus Selector3 : BusSelector  OutputSignals=Aux_tqAct_Nm
  sensor out : Outport
  ctrl out : Outport  Port=2
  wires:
  Bus Creator1/1 -> ctrl out/1
  sensor in/1 -> Bus Selector3/1
  Bus Creator2/1 -> sensor out/1  "AuxMech"
  cmd in/1 -> Bus Selector1/1
  Bus Selector3/1 -> Bus Creator2/1  "<Aux_tqAct_Nm>"
  Bus Selector1/1 -> Bus Creator1/1  "<Aux_pwrMechReq_W>"

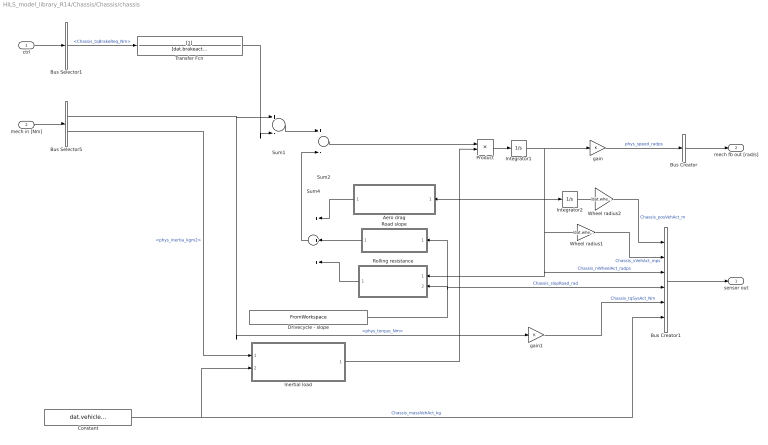
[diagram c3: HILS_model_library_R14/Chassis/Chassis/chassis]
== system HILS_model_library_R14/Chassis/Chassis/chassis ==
  ctrl : Inport
  mech in [Nm] : Inport  Port=2
  Aero drag : Subsystem  Orientation=left
  Bus Creator : BusCreator  Inputs=1
  Bus Creator1 : BusCreator  Inputs=6
  Bus Selector1 : BusSelector  OutputSignals=Chassis_tqBrakeReq_Nm
  Bus Selector5 : BusSelector  OutputSignals=phys_torque_Nm,phys_inertia_kgm2
  Constant : Constant  Value=dat.vehicle.mass.value
  Drivecycle - slope : FromWorkspace  VariableName=[hilsmdl.drivecycle.time.vec, hilsmdl.drivecycle.slope.vec]  SampleTime=0
  Inertial load : Subsystem
  Integrator1 : Integrator  LimitOutput=on  LowerSaturationLimit=0
  Integrator2 : Integrator
  Product : Product  Inputs=*/
  Road slope : Subsystem  Orientation=left
  Rolling resistance : Subsystem  Orientation=left
  Sum1 : Sum  Inputs=+-
  Sum2 : Sum  Inputs=+-
  Sum4 : Sum  Orientation=left  Inputs=+++
  Transfer Fcn : TransferFcn  Denominator=[dat.brakeactuator.timeconstant.value 1]
  Wheel radius1 : Gain  Gain=dat.wheel.radius.value
  Wheel radius2 : Gain  Gain=dat.wheel.radius.value
  gain : Gain
  gain1 : Gain
  sensor out : Outport
  mech fb out [rad/s] : Outport  Port=2
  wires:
  Bus Selector5/2 -> Inertial load/1(Pt inertia)  "<phys_inertia_kgm2>"
  Drivecycle - slope/1 -> Road slope/1(slope1), Bus Creator1/4, Rolling resistance/2(slope)  "Chassis_slopRoad_rad"
  Sum1/1 -> Sum2/1
  Sum4/1 -> Sum2/2
  Aero drag/1(Tq Aero) -> Sum4/1
  Bus Selector1/1 -> Transfer Fcn/1  "<Chassis_tqBrakeReq_Nm>"
  Road slope/1(Tq slope) -> Sum4/2
  Wheel radius1/1 -> Bus Creator1/2  "Chassis_vVehAct_mps"
  gain/1 -> Bus Creator/1  "phys_speed_radps"
  Rolling resistance/1(Tq roll) -> Sum4/3
  Sum2/1 -> Product/1
  Product/1 -> Integrator1/1
  Inertial load/1(Total inertia) -> Product/2
  Integrator2/1 -> Wheel radius2/1
  Integrator1/1 -> Bus Creator1/3, Rolling resistance/1(wheel speed), Wheel radius1/1, Aero drag/1(wheel speed), Integrator2/1, gain/1  "Chassis_nWheelAct_radps"
  ctrl/1 -> Bus Selector1/1
  Bus Creator1/1 -> sensor out/1
  Constant/1 -> Bus Creator1/6, Inertial load/2(mass)  "Chassis_massVehAct_kg"
  mech in [Nm]/1 -> Bus Selector5/1
  Bus Creator/1 -> mech fb out [rad/s]/1
  Bus Selector5/1 -> gain1/1, Sum1/1  "<phys_torque_Nm>"
  Wheel radius2/1 -> Bus Creator1/1  "Chassis_posVehAct_m"
  gain1/1 -> Bus Creator1/5  "Chassis_tqSysAct_Nm"
  Transfer Fcn/1 -> Sum1/2

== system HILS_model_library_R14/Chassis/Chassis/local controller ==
  cmd in : Inport
  sensor in : Inport  Port=2
  Bus Creator1 : BusCreator  Inputs=1
  Bus Creator2 : BusCreator  Inputs=5
  Bus Selector1 : BusSelector  OutputSignals=Chassis_vVehAct_mps,Chassis_nWheelAct_radps,Chassis_massVehAct_kg,Chassis_slopRoad_rad,Chassis_tqSysAct_Nm
  Bus Selector2 : BusSelector  OutputSignals=Chassis_tqBrakeReq_Nm
  sensor out : Outport
  ctrl : Outport  Port=2
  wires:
  Bus Selector1/4 -> Bus Creator2/4  "<Chassis_slopRoad_rad>"
  Bus Selector1/3 -> Bus Creator2/3  "<Chassis_massVehAct_kg>"
  Bus Selector1/2 -> Bus Creator2/2  "<Chassis_nWheelAct_radps>"
  Bus Selector1/1 -> Bus Creator2/1  "<Chassis_vVehAct_mps>"
  cmd in/1 -> Bus Selector2/1
  sensor in/1 -> Bus Selector1/1
  Bus Creator2/1 -> sensor out/1  "Chassis"
  Bus Creator1/1 -> ctrl/1
  Bus Selector2/1 -> Bus Creator1/1  "<Chassis_tqBrakeReq_Nm>"
  Bus Selector1/5 -> Bus Creator2/5  "<Chassis_tqSysAct_Nm>"

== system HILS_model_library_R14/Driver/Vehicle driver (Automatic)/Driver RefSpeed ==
  Chassis_vVehAct_mps : Inport
  Constant1 : Constant  Value=0
  Constant3 : Constant  Value=0
  Data Type Conversion : DataTypeConversion
  Detect Increase1 : simulink/Logic and Bit Operations/Detect Increase  vinit=0.0
  Fcn2 : Fcn  Expr=abs(u)>=0.0001
  From Workspace : FromWorkspace  VariableName=[hilsmdl.drivecycle.time.vec, hilsmdl.drivecycle.speed.vec]  SampleTime=0
  Gain1 : Gain  Gain=-1
  MinMax2 : MinMax  Inputs=2
  MinMax3 : MinMax  Function=max  Inputs=2
  MinMax5 : MinMax  Inputs=2
  PID controller1 : HILS_model_library/Driver/Vehicle driver (Manual)/Driver RefSpeed/PID controller
  Product1 : Product
  Sum2 : Sum  Inputs=-+
  Switch2 : Switch  Threshold=1
  brakes during standstil : simulink/Logic and Bit Operations/Compare To Zero  relop===  LogicOutDataTypeMode=uint8
  resets PI when vehicle starts again1 : simulink/Logic and Bit Operations/Compare To Zero  relop=~=  LogicOutDataTypeMode=uint8
  CycleReferenceSpeed_mps : Outport
  Drv_BrkPedl_rat : Outport  Port=2
  Drv_AccPedl_rat : Outport  Port=3
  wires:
  Switch2/1 -> MinMax3/1, MinMax2/1
  MinMax5/1 -> Switch2/1
  brakes during standstil/1 -> Switch2/2
  Constant3/1 -> MinMax5/2
  resets PI when vehicle starts again1/1 -> Detect Increase1/1
  MinMax3/1 -> Drv_AccPedl_rat/1  "Drv_AccPedl_rat"
  Detect Increase1/1 -> Data Type Conversion/1
  Constant1/1 -> MinMax3/2, MinMax2/2
  Fcn2/1 -> Product1/2
  PID controller1/1 -> Fcn2/1, Product1/1
  Product1/1 -> Switch2/3, MinMax5/1
  From Workspace/1 -> resets PI when vehicle starts again1/1, CycleReferenceSpeed_mps/1, brakes during standstil/1, Sum2/2  "desired vehicle speed"
  Gain1/1 -> Drv_BrkPedl_rat/1  "Drv_BrkPedl_rat"
  MinMax2/1 -> Gain1/1
  Chassis_vVehAct_mps/1 -> Sum2/1
  Sum2/1 -> PID controller1/2
  Data Type Conversion/1 -> PID controller1/1

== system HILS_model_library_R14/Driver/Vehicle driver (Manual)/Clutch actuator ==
  Drv_AccPedl_rat : Inport
  Drv_gearReq : Inport  Port=2
  releaseDrvResetAndHoldZero : Inport  Port=3
  Clutch actuator a : Subsystem
  Clutch actuator b : Subsystem
  Compare To Zero : simulink/Logic and Bit Operations/Compare To Zero  relop=>  LogicOutDataTypeMode=uint8
  Compare To Zero1 : Subsystem  mask(Compare To Zero){relop===, LogicOutDataTypeMode=uint8, ZeroCross=on}
      mask prompts: relop "Operator:"; LogicOutDataTypeMode "Output data type mode:"; ZeroCross "Enable zero-crossing detection"
      mask help: Determine how a signal compares to zero.
      mask init:
      | blkName = gcb;
      | 
      | if strcmp(get_param(gcbh,'LogicOutDataTypeMode'),'boolean')
      | 	setValue = 'Boolean';
      | else
      |     setValue = 'Specify via dialog';
      | end
      | 
      | set_param([blkName,'/Compare'],'relop',relop, ...
      | 	'LogicOutDataTypeMode', setValue, 'ZeroCross', ZeroCross);
  Logical Operator1 : Logic  Operator=OR  AllPortsSameDT=off
  Logical Operator2 : Logic  Operator=OR  AllPortsSameDT=off
  Logical Operator3 : Logic  AllPortsSameDT=off
  Logical Operator4 : Logic  Operator=OR  AllPortsSameDT=off
  Memory : Memory
  S-R Flip-Flop : simulink_extras/Flip Flops/S-R Flip-Flop  initial_condition=0
  S-R Flip-Flop1 : simulink_extras/Flip Flops/S-R Flip-Flop  initial_condition=0
  Terminator : Terminator
  Terminator1 : Terminator
  DrvResetAndHoldZero : Outport
  Drv_gearReq_out : Outport  Port=2
  DrvReqClu : Outport  Port=3
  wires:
  Clutch actuator b/1(Out1) -> DrvReqClu/1
  Logical Operator1/1 -> Clutch actuator b/1(In1)  "DrvReqClu"
  Logical Operator3/1 -> S-R Flip-Flop1/1
  S-R Flip-Flop1/2 -> Terminator1/1
  S-R Flip-Flop1/1 -> Logical Operator2/1
  Compare To Zero/1 -> Logical Operator3/1
  Memory/1 -> Compare To Zero/1
  Drv_AccPedl_rat/1 -> Memory/1
  S-R Flip-Flop/2 -> Terminator/1
  S-R Flip-Flop/1 -> Logical Operator2/2
  Clutch actuator a/2(DrvReqCluGearUp) -> Logical Operator1/2, S-R Flip-Flop/1
  Clutch actuator a/1(DrvReqCluGearDwn) -> Logical Operator3/2, Logical Operator1/1
  Drv_gearReq/1 -> Clutch actuator b/2(In2), Drv_gearReq_out/1, Clutch actuator a/1(Drv_gearReq), Compare To Zero1/1(u)
  releaseDrvResetAndHoldZero/1 -> S-R Flip-Flop1/2, S-R Flip-Flop/2
  Logical Operator2/1 -> Logical Operator4/2
  Logical Operator4/1 -> DrvResetAndHoldZero/1
  Compare To Zero1/1(y) -> Logical Operator4/1

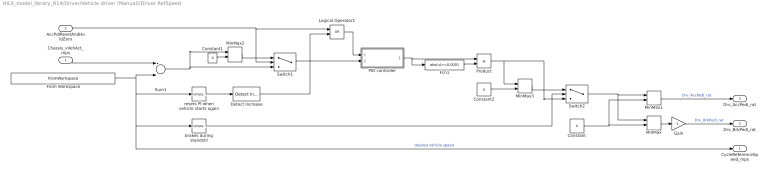
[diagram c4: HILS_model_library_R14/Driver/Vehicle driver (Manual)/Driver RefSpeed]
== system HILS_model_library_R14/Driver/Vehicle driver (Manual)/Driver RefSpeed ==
  Chassis_vVehAct_mps : Inport
  AccPdlResetAndHoldZero : Inport  Port=2
  Constant : Constant  Value=0
  Constant1 : Constant  Value=0
  Constant2 : Constant  Value=0
  Detect Increase : simulink/Logic and Bit Operations/Detect Increase  vinit=0.0
  Fcn1 : Fcn  Expr=abs(u)>=0.0001
  From Workspace : FromWorkspace  VariableName=[hilsmdl.drivecycle.time.vec, hilsmdl.drivecycle.speed.vec]  SampleTime=0
  Gain : Gain  Gain=-1
  Logical Operator1 : Logic  Operator=OR  AllPortsSameDT=off
  MinMax : MinMax  Inputs=2
  MinMax1 : MinMax  Function=max  Inputs=2
  MinMax2 : MinMax  Inputs=2
  MinMax3 : MinMax  Inputs=2
  PID controller : Subsystem
  Product : Product
  Sum1 : Sum  Inputs=-+
  Switch1 : Switch  Criteria=u2 ~= 0
  Switch2 : Switch  Threshold=1
  brakes during standstil : simulink/Logic and Bit Operations/Compare To Zero  relop===  LogicOutDataTypeMode=uint8
  resets PI when vehicle starts again : simulink/Logic and Bit Operations/Compare To Zero  relop=~=  LogicOutDataTypeMode=uint8
  CycleReferenceSpeed_mps : Outport
  Drv_BrkPedl_rat : Outport  Port=2
  Drv_AccPedl_rat : Outport  Port=3
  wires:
  Switch2/1 -> MinMax1/1, MinMax/1
  MinMax3/1 -> Switch2/1
  brakes during standstil/1 -> Switch2/2
  Constant2/1 -> MinMax3/2
  resets PI when vehicle starts again/1 -> Detect Increase/1
  MinMax1/1 -> Drv_AccPedl_rat/1  "Drv_AccPedl_rat"
  Logical Operator1/1 -> PID controller/1(PI reset)
  Constant/1 -> MinMax1/2, MinMax/2
  Fcn1/1 -> Product/2
  PID controller/1(PI output) -> Fcn1/1, Product/1
  Product/1 -> Switch2/3, MinMax3/1
  From Workspace/1 -> Sum1/2, resets PI when vehicle starts again/1, CycleReferenceSpeed_mps/1, brakes during standstil/1  "desired vehicle speed"
  Gain/1 -> Drv_BrkPedl_rat/1  "Drv_BrkPedl_rat"
  MinMax/1 -> Gain/1
  Chassis_vVehAct_mps/1 -> Sum1/1
  Constant1/1 -> MinMax2/2
  MinMax2/1 -> Switch1/1
  Switch1/1 -> PID controller/2(PI input)
  Sum1/1 -> Switch1/3, MinMax2/1
  AccPdlResetAndHoldZero/1 -> Switch1/2, Logical Operator1/1
  Detect Increase/1 -> Logical Operator1/2
